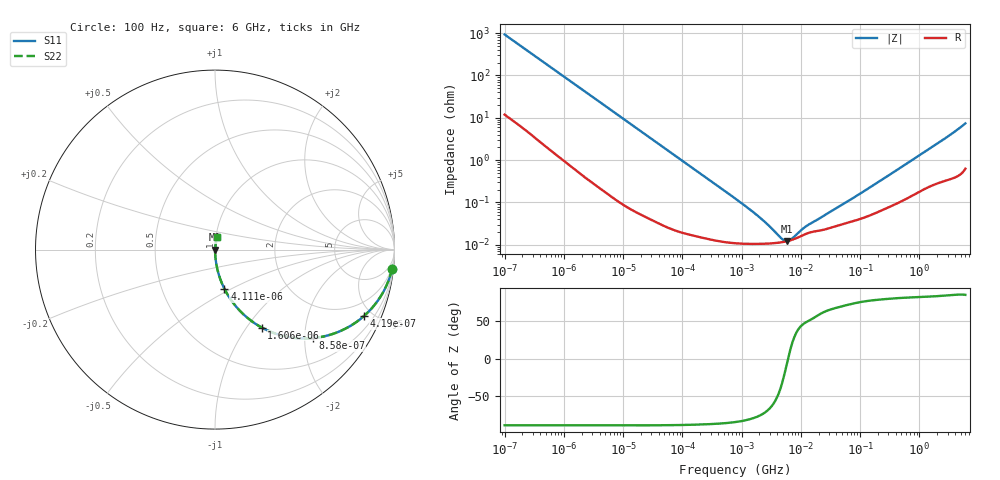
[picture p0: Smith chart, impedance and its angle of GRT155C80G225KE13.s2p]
!Murata Part Number: GRT155C80G225KE13
!These Parameters are Measured in Series Mode Connection
!Data Generated on Jun 19, 2026
!  o--ll--o
!Port1  Port2
!  o------o
!Operation Temp=25[degC], DC Bias Voltage=0[V]
!Freq. Start=100[Hz] Stop=6[GHz] 401[Steps]
# Hz S RI R 50
!Freq.(Hz) S11(Real) S11(Imag) S21(Real) S21(Imag) S12(Real) S12(Imag) S22(Real) S22(Imag)
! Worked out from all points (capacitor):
!   401 points, 100 Hz to 6 GHz, reference 50 ohm
!   read as one part in series: C = 1.71 uF near 109 Hz
!   lowest |Z| = 12.2 mohm at 5.809 MHz (marker M1)
!   series resonance near 6.101 MHz, so ESL is about 400 pH
!   S11 on the Smith chart (normalised r, x): 100 Hz: 1, -19; 419 Hz: 1.05, -4.48; 858 Hz: 1.02, -2.20; 1.606 kHz: 1.01, -1.18; 4.111 kHz: 1.00, -0.46; 6 GHz: 1.01, +0.15
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100  0.9872 -0.1061  0.0128 0.1061  0.0128 0.1061  0.9872 -0.1061
224  0.9433 -0.2252  0.0567 0.2252  0.0567 0.2252  0.9433 -0.2252
419  0.8314 -0.3688  0.1686 0.3688  0.1686 0.3688  0.8314 -0.3688
600  0.7097 -0.4486  0.2903 0.4486  0.2903 0.4486  0.7097 -0.4486
858  0.5474 -0.4926  0.4526 0.4926  0.4526 0.4926  0.5474 -0.4926
1174  0.3949 -0.4839  0.6051 0.4839  0.6051 0.4839  0.3949 -0.4839
1606  0.2605 -0.4341  0.7395 0.4341  0.7395 0.4341  0.2605 -0.4341
2008  0.1849 -0.3835  0.8151 0.3835  0.8151 0.3835  0.1849 -0.3835
2873  0.1009 -0.2966  0.8991 0.2966  0.8991 0.2966  0.1009 -0.2966
4111  0.0528 -0.2191  0.9472 0.2191  0.9472 0.2191  0.0528 -0.2191
11009  0.0083 -0.0862  0.9917 0.0862  0.9917 0.0862  0.0083 -0.0862
40335  0.000888 -0.0239  0.9991 0.0239  0.9991 0.0239  0.000888 -0.0239
774597  0.000111 -0.00125  0.9999 0.00125  0.9999 0.00125  0.000111 -0.00125
2169299  0.000106 -0.000395  0.9999 0.000395  0.9999 0.000395  0.000106 -0.000395
4643984  0.000114 -8.77e-05  0.9999 8.77e-05  0.9999 8.77e-05  0.000114 -8.77e-05
5809218  0.000121 -1.54e-05  0.9999 1.54e-05  0.9999 1.54e-05  0.000121 -1.54e-05
6948629  0.00013 4.05e-05  0.9999 -4.05e-05  0.9999 -4.05e-05  0.00013 4.05e-05
1.087309e7  0.000169 0.000173  0.9998 -0.000173  0.9998 -0.000173  0.000169 0.000173
1.555665e7  0.000202 0.000268  0.9998 -0.000268  0.9998 -0.000268  0.000202 0.000268
3.124326e8  0.000803 0.0044  0.9992 -0.0044  0.9992 -0.0044  0.000803 0.0044
1.95892e9  0.00332 0.0236  0.9967 -0.0236  0.9967 -0.0236  0.00332 0.0236
6e9  0.0115 0.0722  0.9885 -0.0722  0.9885 -0.0722  0.0115 0.0722
